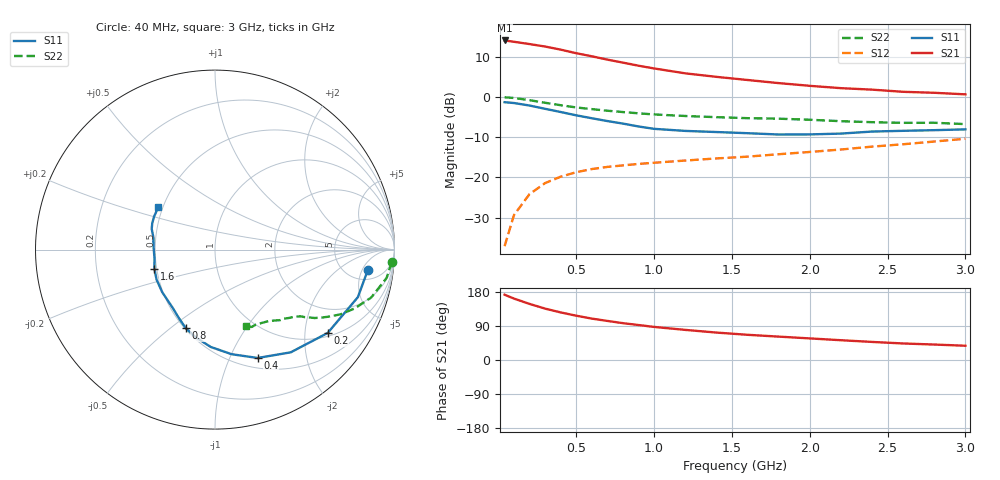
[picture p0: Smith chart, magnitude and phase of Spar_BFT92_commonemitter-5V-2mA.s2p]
! Filename:  BFT92A.S2P  Version:  2.0
! NXP part #: BFT92  Date: May 1990
! Bias condition: Vce=-5V, Ic=-2mA
#  MHz  S  MA  R  50
! Freq  S11  S21  S12  S22  !GUM [dB]
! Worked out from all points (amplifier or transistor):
!   21 points, 40 MHz to 3 GHz, reference 50 ohm
!   highest |S21| = 14.0 dB at 40 MHz (marker M1)
!   |S21| within 3 dB of that: start of sweep to 481.1 MHz
!   unconditionally stable (mu >= 1): 1.48 GHz to end of sweep
!   at 300 MHz: K = 0.33, MSG = 17.0 dB, |S12| = -21.4 dB
!   at 1 GHz: K = 0.83, MSG = 11.7 dB, |S12| = -16.4 dB
!   at 3 GHz: K = 1.02, MAG = 4.6 dB, |S12| = -10.4 dB
!   S11 on the Smith chart (normalised r, x): 40 MHz: 7.49, -6.50; 200 MHz: 1.10, -2.62; 400 MHz: 0.61, -1.28; 800 MHz: 0.51, -0.56; 1.6 GHz: 0.49, -0.12; 3 GHz: 0.47, +0.26
40  0.859 -7.6  5.019 172.2  0.014 84.9  0.988 -4.0
100  0.839 -18.4  4.831 162.1  0.034 78.5  0.969 -9.4
200  0.781 -36.5  4.528 148.0  0.062 69.2  0.91 -17.1
300  0.711 -53.6  4.217 135.6  0.085 62.0  0.845 -22.8
400  0.649 -68.5  3.862 125.6  0.102 57.0  0.788 -27.2
500  0.59 -81.0  3.485 116.9  0.116 53.5  0.739 -30.3
600  0.543 -92.5  3.192 109.3  0.127 51.0  0.705 -32.5
700  0.501 -102.2  2.901 103.1  0.135 49.5  0.673 -34.5
800  0.466 -110.6  2.664 97.2  0.141 48.5  0.648 -35.7
900  0.429 -118.4  2.438 92.3  0.147 48.0  0.625 -37.0
1000  0.401 -126.0  2.255 87.3  0.152 47.9  0.605 -37.9
1200  0.378 -141.0  1.961 79.5  0.162 48.1  0.579 -40.3
1400  0.366 -152.8  1.773 72.4  0.172 49.5  0.56 -42.9
1600  0.354 -162.6  1.621 66.5  0.181 51.8  0.544 -45.0
1800  0.341 -171.1  1.483 61.7  0.194 54.1  0.536 -47.1
2000  0.342 178.0  1.372 57.0  0.207 55.9  0.52 -49.4
2200  0.35 168.7  1.283 52.2  0.222 57.7  0.499 -52.8
2400  0.371 161.9  1.23 47.7  0.241 58.9  0.485 -57.3
2600  0.379 157.3  1.156 43.6  0.258 59.9  0.476 -61.5
2800  0.386 151.7  1.124 40.8  0.279 61.1  0.477 -64.7
3000  0.395 143.2  1.075 37.6  0.302 61.5  0.459 -67.8
